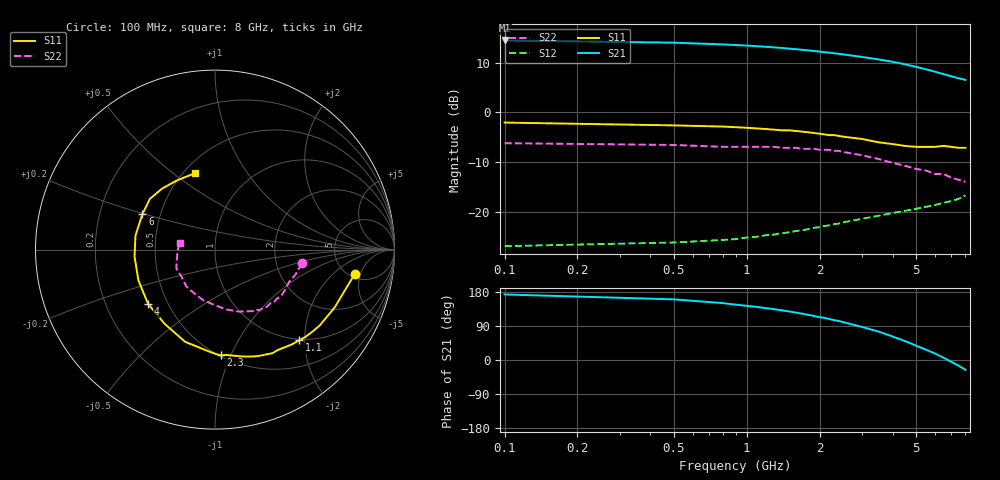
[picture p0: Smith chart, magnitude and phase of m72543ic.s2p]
!  MGA-72543 S PARAMETERS
!  Vd=3V  Id=10 mA Vc=0.6V  LAST UPDATED 01-27-99
# ghz s ma r 50
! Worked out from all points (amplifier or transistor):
!   31 points, 100 MHz to 8 GHz, reference 50 ohm
!   highest |S21| = 14.5 dB at 100 MHz (marker M1)
!   |S21| within 3 dB of that: start of sweep to 2.685 GHz
!   unconditionally stable (mu >= 1): start of sweep to end of sweep
!   at 1.1 GHz: K = 1.11, MAG = 17.1 dB, |S12| = -25.0 dB
!   at 2.1 GHz: K = 1.09, MAG = 15.6 dB, |S12| = -22.9 dB
!   at 8 GHz: K = 1.33, MAG = 8.2 dB, |S12| = -16.7 dB
!   lowest NFmin = 1.33 dB at 800 MHz
!   S11 on the Smith chart (normalised r, x): 100 MHz: 5.52, -4.03; 1.1 GHz: 0.98, -1.89; 2.3 GHz: 0.51, -0.92; 4 GHz: 0.39, -0.31; 6 GHz: 0.40, +0.20; 8 GHz: 0.57, +0.60
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0.1  0.79 -10.0  5.302 173.0  0.045 19.0  0.49 -9.0
0.5  0.74 -26.0  5.037 160.0  0.049 13.0  0.47 -17.0
0.8  0.72 -36.0  4.836 150.0  0.052 15.0  0.45 -24.0
0.9  0.71 -40.0  4.77 146.0  0.053 16.0  0.45 -27.0
1.1  0.69 -47.0  4.641 140.0  0.056 17.0  0.45 -31.0
1.4  0.66 -58.0  4.452 131.0  0.061 19.0  0.44 -38.0
1.6  0.65 -64.0  4.328 125.0  0.064 19.0  0.44 -42.0
1.9  0.62 -74.0  4.149 116.0  0.069 18.0  0.43 -48.0
2.1  0.6 -80.0  4.039 111.0  0.072 18.0  0.42 -52.0
2.3  0.59 -87.0  3.938 105.0  0.075 17.0  0.41 -55.0
2.4  0.58 -90.0  3.889 103.0  0.076 16.0  0.41 -57.0
3  0.54 -108.0  3.616 87.0  0.085 13.0  0.37 -69.0
3.5  0.5 -124.0  3.419 75.0  0.091 9.0  0.34 -79.0
4  0.48 -141.0  3.234 62.0  0.097 6.0  0.31 -90.0
4.5  0.46 -158.0  3.054 50.0  0.102 2.0  0.29 -103.0
5  0.45 -175.0  2.875 38.0  0.107 -3.0  0.27 -115.0
5.5  0.45 170.0  2.718 27.0  0.112 -6.0  0.26 -128.0
6  0.45 154.0  2.567 17.0  0.117 -10.0  0.24 -141.0
6.5  0.46 142.0  2.43 6.0  0.123 -14.0  0.24 -154.0
7  0.45 131.0  2.31 -5.0  0.128 -19.0  0.22 -165.0
7.5  0.44 119.0  2.206 -15.0  0.135 -23.0  0.21 -176.0
8  0.44 105.0  2.125 -26.0  0.146 -28.0  0.2 169.0
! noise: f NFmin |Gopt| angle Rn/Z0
0.8  1.33  0.45  37  0.23
1  1.34  0.38  42  0.24
1.8  1.44  0.25  56  0.23
2  1.47  0.24  62  0.22
2.2  1.49  0.23  68  0.21
2.4  1.51  0.22  74  0.2
3  1.55  0.2  92  0.19
4  1.58  0.17  131  0.15
5  1.62  0.19  177  0.13
6  1.67  0.25  -136  0.15
